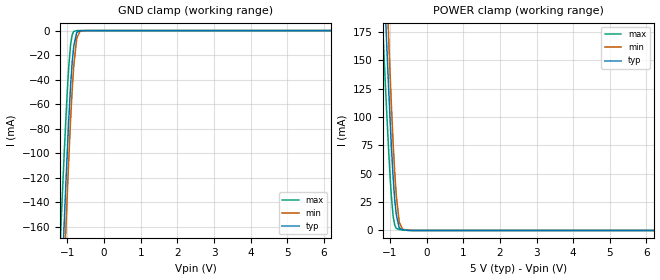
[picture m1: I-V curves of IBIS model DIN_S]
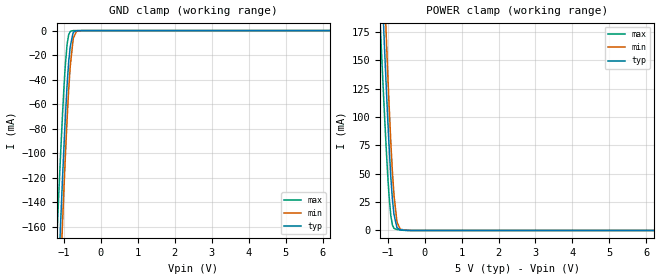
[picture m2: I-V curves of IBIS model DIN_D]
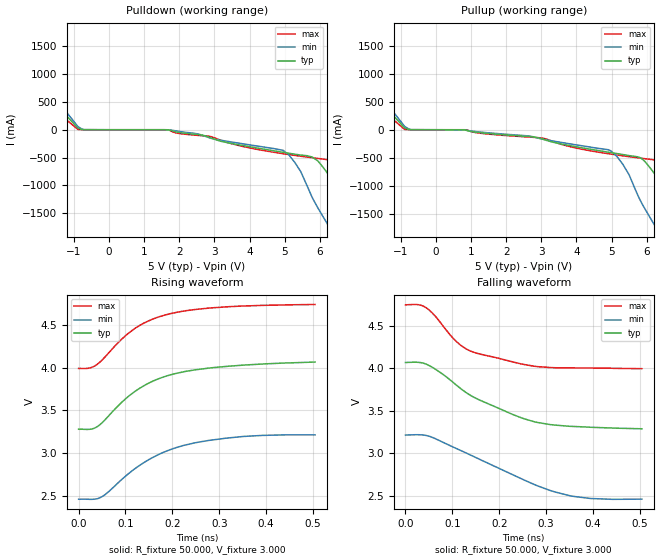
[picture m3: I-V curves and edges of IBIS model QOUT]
|Texas Instruments Incorporated
|5V  PECL/ECL 1:2 Fanout Buffer
|Valid for clock frequencies upto 3.4 - 3.5GHz
|*_S components are valid for parts used with D and DB in Single-Ended mode
|*_D components are valid for parts used with D and DB in Differential mode
| Marketing part#   Voltage Range   Package-type   #pins
|SN65EL16D   4.2V-5.7V   SOIC   8-pin
|SN65EL16DGK   4.2V-5.7V   MSOP(SOIC-TSSOP)   8-pin
[IBIS Ver]   4.0
[File name]   sn65el16.ibs
[File Rev]   1.0
[Date]   02/02/2009
[Source]   Texas Instruments Incorporated.
   Analog-eLab, HPA
   12500 TI Blvd
   Dallas, TX -75243
   For Support e-mail: elab_ibis@list.ti.com
[Notes]   Revision History:
   1.0: 02/02/2009
   - Model based on Simulations in TISPICE
   - Model not matched to silicon measurements
   - Separate Models and components with D/DB configured
   as single-ended and differential
[Disclaimer]
 This product is designed as an aid for customers of Texas Instruments.
 No warranties, either expressed or implied, with respect to this third
 party software (if any) or with respect to its fitness for any
 particular purpose is claimed by Texas Instruments or the author. The
 software (if any) is provided solely on an "as is" basis. The entire
 risk as to its quality and performance is with the customer
[Copyright] (C) Copyright 2009 Texas Instruments Incorporated.
   All rights reserved.
|   SN65EL16D_S with D/DB configured as single-ended
[Component]   SN65EL16D_S
[Manufacturer]  Texas Instruments Incorporated
[Package]   |8-pin SOIC
|   typ   min   max
R_pkg   0.347   0.243   0.450
L_pkg   2.091nH   1.865nH   2.317nH
C_pkg   0.417pF   0.391pF   0.444pF
[Pin]   signal_name   model_name   R_pin   L_pin   C_pin
1   NC   NC   0.03861   1.24238nH   0.38967pF
2   D   DIN_S   0.45016   2.31200nH   0.39081pF
3   DB   DIN_S   0.45022   2.31675nH   0.39335pF
4   VBB   NC   0.41536   2.47060nH   0.46537pF
5   VEE   GND   0.41551   2.47564nH   0.46746pF
6   QB   QOUT   0.24315   1.88180nH   0.44358pF
7   Q   QOUT   0.24302   1.86517nH   0.44219pF
8   VCC   POWER   0.41552   2.46732nH   0.46672pF
|   SN65EL16DGK_S with D/DB configured as single-ended
[Component]   SN65EL16DGK_S
[Manufacturer]  Texas Instruments Incorporated
[Package]   |8-pin SOIC-TSSOP(MSOP)
|   typ   min   max
R_pkg   0.265   0.190   0.340
L_pkg   1.571nH   1.446nH   1.696nH
C_pkg   0.420pF   0.403pF   0.438pF
[Pin]   signal_name   model_name   R_pin   L_pin   C_pin
1   NC   NC   0.03760   0.74741nH   0.31231pF
2   D   DIN_S   0.34015   1.69514nH   0.40289pF
3   DB   DIN_S   0.34015   1.69570nH   0.40558pF
4   VBB   NC   0.36621   1.80969nH   0.38808pF
5   VEE   GND   0.36621   1.80971nH   0.38874pF
6   QB   QOUT   0.18959   1.44751nH   0.43796pF
7   Q   QOUT   0.18959   1.44613nH   0.43787pF
8   VCC   POWER   0.36621   1.80560nH   0.38855pF
[Diff_pin]   inv_pin   vdiff   tdelay_typ   tdelay_min   tdelay_max
| The '7' pin is Diff_pin and the '6' pin is inv_pin
7   6   0.300   0   NA   NA
|   SN65EL16D_D with D/DB configured as Differential
[Component]   SN65EL16D_D
[Manufacturer]  Texas Instruments Incorporated
[Package]   |8-pin SOIC
|   typ   min   max
R_pkg   0.347   0.243   0.450
L_pkg   2.091nH   1.865nH   2.317nH
C_pkg   0.417pF   0.391pF   0.444pF
[Pin]   signal_name   model_name   R_pin   L_pin   C_pin
1   NC   NC   0.03861   1.24238nH   0.38967pF
2   D   DIN_D   0.45016   2.31200nH   0.39081pF
3   DB   DIN_D   0.45022   2.31675nH   0.39335pF
4   VBB   NC   0.41536   2.47060nH   0.46537pF
5   VEE   GND   0.41551   2.47564nH   0.46746pF
6   QB   QOUT   0.24315   1.88180nH   0.44358pF
7   Q   QOUT   0.24302   1.86517nH   0.44219pF
8   VCC   POWER   0.41552   2.46732nH   0.46672pF
|   SN65EL16DGK_D with D/DB configured as Differential
[Component]   SN65EL16DGK_D
[Manufacturer]  Texas Instruments Incorporated
[Package]   |8-pin SOIC-TSSOP(MSOP)
|   typ   min   max
R_pkg   0.265   0.190   0.340
L_pkg   1.571nH   1.446nH   1.696nH
C_pkg   0.420pF   0.403pF   0.438pF
[Pin]   signal_name   model_name   R_pin   L_pin   C_pin
1   NC   NC   0.03760   0.74741nH   0.31231pF
2   D   DIN_D   0.34015   1.69514nH   0.40289pF
3   DB   DIN_D   0.34015   1.69570nH   0.40558pF
4   VBB   NC   0.36621   1.80969nH   0.38808pF
5   VEE   GND   0.36621   1.80971nH   0.38874pF
6   QB   QOUT   0.18959   1.44751nH   0.43796pF
7   Q   QOUT   0.18959   1.44613nH   0.43787pF
8   VCC   POWER   0.36621   1.80560nH   0.38855pF
[Diff_pin]   inv_pin   vdiff   tdelay_typ   tdelay_min   tdelay_max
| The '2,7' pins are Diff_pin(s) and the '3,6' pins are inv_pin(s)
2   3   0.750   0   NA   NA
7   6   0.300   0   NA   NA
| Models and submodels in the file (3): DIN_S (Input_ECL), DIN_D (Input_ECL), QOUT (Output_ECL)
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|   DIN_S Input_ECL MODEL with D/DB configured as Differential
[Model]   DIN_S
Model_type   Input_ECL
|Signals   D & DB pair  for 3.3V option
|Input Levels
Vinl = 3.3575V
Vinh = 3.9775V
|   typ   min   max
C_comp   0.3757pF   0.4341pF   0.3313pF
[Model Spec]
Vinl   3.3575V   3.190V   3.525V
Vinh   3.9775V   3.835V   4.120V
[Voltage Range]   5.0V   4.2V   5.7V
| Junction Temperature (Ambient temp is 25C typ, 85C min,  -40C max)
[Temperature Range]   40.0   100.0   -40.0
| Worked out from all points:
|   GND clamp passes 1 mA (typ) near -0.72 V on its own axis
|   POWER clamp passes 1 mA (typ) near -0.68 V on its own axis
[GND Clamp]
|   Voltage   I(typ)   I(min)   I(max)
-5V       -3.652A    -3.933A    -3.241A
-1.231V   -264mA     -312.3mA   -196.7mA
-1.173V   -218.9mA   -263.7mA   -156mA
-1.111V   -172.6mA   -213.6mA   -114.3mA
-1.087V   -155mA     -194.6mA   -98.62mA
-1.037V   -119.7mA   -156.3mA   -67.58mA
-962.4mV  -71.43mA   -103.3mA   -28.43mA
-914.5mV  -44.58mA   -72.39mA   -11.23mA
-828.4mV  -12.78mA   -29.02mA   -685.3uA
-742.4mV  -1.259mA   -5.907mA   -23.96uA
-515.6mV  -34.71uA   -15.81uA   -10.43uA
10V       0A         0A         0A
[POWER Clamp]
|   Voltage   I(typ)   I(min)   I(max)
-5V       3.68A      4.765A     3.126A
-1.231V   276.9mA    346.5mA    203.2mA
-1.173V   229.5mA    291.1mA    161.6mA
-1.111V   180.8mA    234.4mA    118.8mA
-1.037V   125.3mA    170mA      70.66mA
-962.4mV  74.81mA    111.2mA    30.5mA
-914.5mV  46.93mA    77.4mA     12.89mA
-828.4mV  14.09mA    30.97mA    1.902mA
-751.6mV  2.83mA     8.414mA    859.4uA
-656.3mV  567.6uA    1.14mA     454.6uA
-397.6mV  25.28uA    70.89uA    11.71uA
10V       0A         0A         0A
|   DIN_D Input_ECL MODEL with D/DB configured as Differential
[Model]   DIN_D
Model_type   Input_ECL
|Signals   D & DB pair  for 3.3V option
|Input Levels
Vinl = 2.80V
Vinh = 3.55V
|   typ   min   max
C_comp   0.3757pF   0.4341pF   0.3313pF
[Model Spec]
Vinl   2.80V   1.75V   3.85V
Vinh   3.55V   2.50V   4.60V
[Voltage Range]   5.0V   4.2V   5.7V
| Junction Temperature (Ambient temp is 25C typ, 85C min,  -40C max)
[Temperature Range]   40.0   100.0   -40.0
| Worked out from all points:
|   GND clamp passes 1 mA (typ) near -0.72 V on its own axis
|   POWER clamp passes 1 mA (typ) near -0.68 V on its own axis
[GND Clamp]
|   Voltage   I(typ)   I(min)   I(max)
-5V       -3.652A    -3.933A    -3.241A
-1.231V   -264mA     -312.3mA   -196.7mA
-1.173V   -218.9mA   -263.7mA   -156mA
-1.111V   -172.6mA   -213.6mA   -114.3mA
-1.087V   -155mA     -194.6mA   -98.62mA
-1.037V   -119.7mA   -156.3mA   -67.58mA
-962.4mV  -71.43mA   -103.3mA   -28.43mA
-914.5mV  -44.58mA   -72.39mA   -11.23mA
-828.4mV  -12.78mA   -29.02mA   -685.3uA
-742.4mV  -1.259mA   -5.907mA   -23.96uA
-515.6mV  -34.71uA   -15.81uA   -10.43uA
10V       0A         0A         0A
[POWER Clamp]
|   Voltage   I(typ)   I(min)   I(max)
-5V       3.68A      4.765A     3.126A
-1.231V   276.9mA    346.5mA    203.2mA
-1.173V   229.5mA    291.1mA    161.6mA
-1.111V   180.8mA    234.4mA    118.8mA
-1.037V   125.3mA    170mA      70.66mA
-962.4mV  74.81mA    111.2mA    30.5mA
-914.5mV  46.93mA    77.4mA     12.89mA
-828.4mV  14.09mA    30.97mA    1.902mA
-751.6mV  2.83mA     8.414mA    859.4uA
-656.3mV  567.6uA    1.14mA     454.6uA
-397.6mV  25.28uA    70.89uA    11.71uA
10V       0A         0A         0A
|   QOUT Output_ECL MODEL
[Model]   QOUT
Model_type   Output_ECL
| Signals   Q0/Q0B and Q1/Q1B pair  for 3.3V option
Cref = 0.0pF   |Timing specification test load capacitance value
Rref = 50.00Ohm
| variable   typ   min   max
C_comp   0.4296pF   0.4336pF   0.3427pF
[Model Spec]
Vref   3.0V   2.2V   3.7V
Vmeas   3.0V   2.2V   3.7V
[pullup reference]   5.0V   4.2V   5.7V
[pulldown reference]   5.0V   4.2V   5.7V
| Junction Temperature (Ambient temp is 25C typ, 85C min,  -40C max)
[Temperature Range]   40.0   100.0   -40.0
[Voltage range]   5.0V   4.2V   5.7V
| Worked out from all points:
|   rising waveform, R_fixture 50.000, V_fixture 3.000: 20-80 % time 127ps typ, 131ps min, 110ps max; typ from 3.28 V to 4.07 V
|   falling waveform, R_fixture 50.000, V_fixture 3.000: 20-80 % time 151ps typ, 179ps min, 110ps max; typ from 4.07 V to 3.29 V
[Pulldown]
|   Voltage   I(typ)   I(min)   I(max)
-5V       3.639A     4.729A     3.081A
-3.585V   2.358A     3.016A     1.987A
-2.677V   1.542A     1.941A     1.289A
-884.6mV  31.32mA    57.53mA    5.304mA
4.952V    -405.6mA   -370.1mA   -431.6mA
6.415V    -984.5mA   -1.912A    -550.7mA
7.318V    -1.898A    -2.908A    -1.101A
8.195V    -2.802A    -3.948A    -1.888A
9.183V    -3.878A    -2.725A    -2.812A
9.292V    -4.006A    -159.4mA   -2.915A
9.764V    -4.571A    31.09A     -3.351A
10V       -3.272A    64.25A     -3.58A
[Pullup]
|   Voltage   I(typ)   I(min)   I(max)
-5V       3.639A     4.729A     3.081A
-3.316V   2.116A     2.695A     1.779A
-2.677V   1.542A     1.941A     1.289A
-884.6mV  31.32mA    57.53mA    5.304mA
4.985V    -408.7mA   -379.4mA   -435.3mA
5.815V    -499.7mA   -1.259A    -506.9mA
6.36V     -917.5mA   -1.852A    -552.7mA
7.329V    -1.925A    -2.921A    -1.136A
8.299V    -2.938A    -4.083A    -1.993A
9.184V    -3.882A    -5.157A    -2.815A
9.828V    -3.345A    16.13A     -3.413A
10V       642.9mA    34.28A     -3.577A
[Ramp]
R_load = 50.00Ohm
|   typ   min   max
dV/dt_r   452.282mV/127.189ps 393.774mV/131.728ps 449.692mV/110.196ps
dV/dt_f   468.903mV/151.294ps 404.770mV/179.559ps 451.149mV/110.044ps
[Rising Waveform]
R_fixture = 50.000
V_fixture = 3.000
V_fixture_min = 2.200
V_fixture_max = 3.700
|  time   V(typ)   V(min)   V(max)
0s        3.278V     2.457V     3.991V
27.02ps   3.28V      2.456V     4.002V
49.82ps   3.353V     2.487V     4.088V
91.27ps   3.59V      2.685V     4.331V
120ps     3.721V     2.815V     4.46V
179.6ps   3.888V     3.004V     4.61V
226.8ps   3.955V     3.092V     4.666V
309.5ps   4.012V     3.17V      4.711V
393ps     4.043V     3.206V     4.731V
504.4ps   4.066V     3.212V     4.741V
[Falling Waveform]
R_fixture = 50.000
V_fixture = 3.000
V_fixture_min = 2.200
V_fixture_max = 3.700
|  time   V(typ)   V(min)   V(max)
0s        4.067V     3.212V     4.746V
27.02ps   4.069V     3.216V     4.748V
44.91ps   4.046V     3.206V     4.709V
76.9ps    3.939V     3.135V     4.52V
116.8ps   3.764V     3.033V     4.274V
156.1ps   3.63V      2.932V     4.17V
274.7ps   3.369V     2.63V      4.023V
351.2ps   3.315V     2.497V     4.003V
394.2ps   3.304V     2.465V     4.002V
504.4ps   3.286V     2.457V     3.994V
